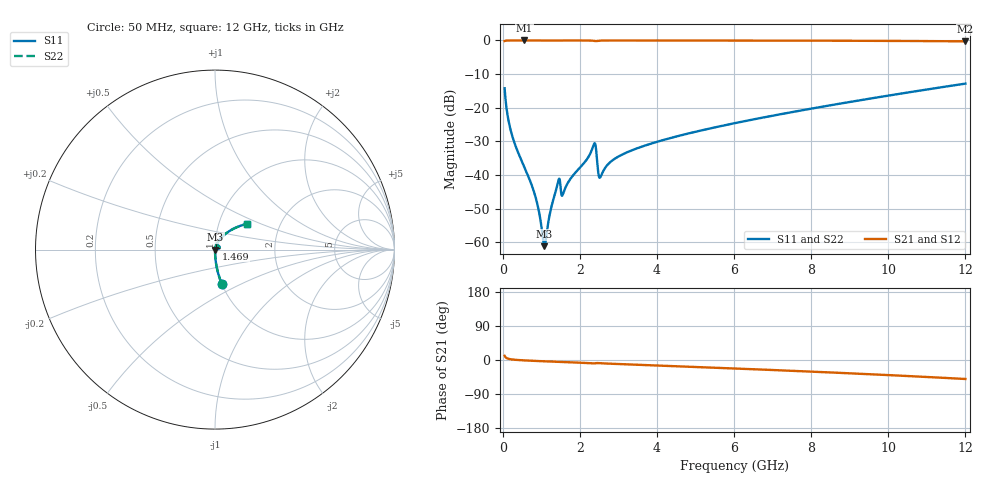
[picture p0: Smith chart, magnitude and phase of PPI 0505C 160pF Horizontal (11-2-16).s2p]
# MHz S MA R 50
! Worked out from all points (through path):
!   1601 points, 50 MHz to 12 GHz, reference 50 ohm
!   highest |S21| = -0.01 dB at 557.9 MHz (marker M1); lowest = -0.3 dB at 12 GHz (marker M2)
!   group delay of S21, straight-line fit = 11.6 ps
!   lowest |S11| = -61.2 dB at 1.081 GHz (marker M3), VSWR 1.00, Z = 50.1 - j0.0135 ohm
!   |S11| at or under -10 dB: start of sweep to end of sweep
!   |S22| runs from -61.2 to -12.8 dB; largest |S21 - S12| = 0
!   S11 on the Smith chart (normalised r, x): 50 MHz: 1.00, -0.40; 1.469 GHz: 1.01, +0.01; 12 GHz: 1.36, +0.41
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50  0.1944 -78.9  0.9807 11.0  0.9807 11.0  0.1944 -78.9
147.0938  0.06616 -86.3  0.9974 3.3  0.9974 3.3  0.06616 -86.3
229.25  0.04142 -87.7  0.9987 1.6  0.9987 1.6  0.04142 -87.7
557.875  0.01328 -88.3  0.9992 -1.0  0.9992 -1.0  0.01328 -88.3
856.625  0.004592 -82.8  0.9992 -2.5  0.9992 -2.5  0.004592 -82.8
1080.688  0.0008731 -8.9  0.9991 -3.4  0.9991 -3.4  0.0008731 -8.9
1125.5  0.001149 35.3  0.999 -3.6  0.999 -3.6  0.001149 35.3
1312.219  0.004287 70.6  0.9988 -4.4  0.9988 -4.4  0.004287 70.6
1424.25  0.007346 67.0  0.9976 -4.9  0.9976 -4.9  0.007346 67.0
1469.062  0.008812 49.4  0.9948 -5.1  0.9948 -5.1  0.008812 49.4
1573.625  0.00538 64.3  0.998 -5.3  0.998 -5.3  0.00538 64.3
2044.156  0.01365 76.4  0.9983 -7.3  0.9983 -7.3  0.01365 76.4
2357.844  0.02791 55.1  0.9873 -9.0  0.9873 -9.0  0.02791 55.1
2402.656  0.02844 29.0  0.9772 -8.7  0.9772 -8.7  0.02844 29.0
2492.281  0.009694 25.9  0.9918 -8.3  0.9918 -8.3  0.009694 25.9
2537.094  0.009338 50.4  0.995 -8.5  0.995 -8.5  0.009338 50.4
2970.281  0.01834 74.4  0.998 -10.5  0.998 -10.5  0.01834 74.4
4038.312  0.03152 72.4  0.9976 -14.6  0.9976 -14.6  0.03152 72.4
6025  0.05898 65.7  0.9959 -22.4  0.9959 -22.4  0.05898 65.7
8019.156  0.09721 57.8  0.9923 -30.7  0.9923 -30.7  0.09721 57.8
10013.31  0.1516 49.0  0.9847 -39.9  0.9847 -39.9  0.1516 49.0
12000  0.2279 38.9  0.969 -50.1  0.969 -50.1  0.2279 38.9
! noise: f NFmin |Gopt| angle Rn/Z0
50  0.0003617  0.8549  0.2997  0.0005325
1372  0.004397  0.7  4.362  0.002865
2701  0.007704  0.6697  8.548  0.004461
4031  0.008262  0.5697  12.52  0.003432
5360  0.01025  0.5479  16.45  0.003966
6682  0.01231  0.5369  20.26  0.00457
8012  0.01447  0.5329  23.98  0.005253
9341  0.01679  0.5347  27.59  0.006047
1.067e+04  0.01933  0.5417  31.09  0.006997
1.2e+04  0.02219  0.5533  34.5  0.008166
